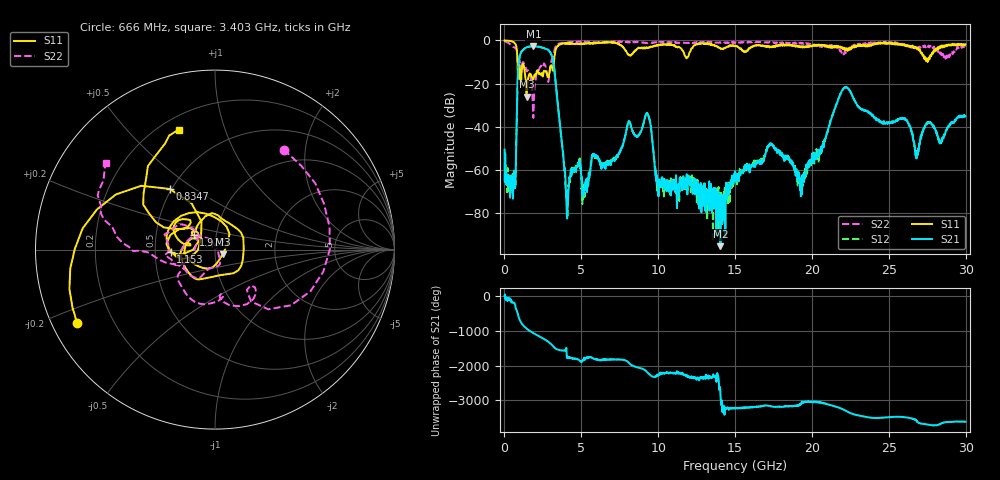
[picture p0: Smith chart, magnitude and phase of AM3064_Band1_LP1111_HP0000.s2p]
# Hz S DB R 50.0
!freq dBS11 angS11 dBS21 angS21 dBS12 angS12 dBS22 angS22
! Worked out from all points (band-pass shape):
!   1600 points, 10 MHz to 29.98 GHz, reference 50 ohm
!   highest |S21| = -2.65 dB at 1.884 GHz (marker M1); lowest = -95.4 dB at 14.05 GHz (marker M2)
!   |S21| within 3 dB of the highest: 1.07 GHz to 2.984 GHz (1.914 GHz wide, 94.4 % of centre)
!   lowest |S11| = -26.1 dB at 1.435 GHz (marker M3), VSWR 1.10, Z = 54.4 - j2.68 ohm
!   |S11| at or under -10 dB: 849 MHz to 3.217 GHz (2.368 GHz wide, 116 % of centre)
!   |S22| runs from -36.0 to -0.2 dB; largest |S21 - S12| = 0.014
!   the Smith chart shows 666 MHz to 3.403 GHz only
!   S11 on the Smith chart (normalised r, x): 666 MHz: 0.07, -0.25; 834.7 MHz: 0.49, +0.40; 1.153 GHz: 0.60, -0.01; 1.922 GHz: 0.78, +0.13; 3.403 GHz: 0.27, +0.71
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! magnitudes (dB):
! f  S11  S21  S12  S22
! 10 MHz  0.0  -50.7  -65.0  -0.2
! 666 MHz  -1.2  -64.3  -66.5  -3.4
! 834.7 MHz  -7.5  -24.9  -24.8  -7.0
! 1.153 GHz  -12.2  -4.9  -4.8  -10.8
! 1.435 GHz  -26.1  -3.2  -3.2  -14.2
! 1.884 GHz  -17.9  -2.7  -2.7  -36.0
! 1.922 GHz  -16.9  -2.7  -2.6  -25.6
! 3.009 GHz  -11.7  -5.9  -5.9  -10.9
! 3.403 GHz  -3.1  -24.9  -25.0  -2.2
! 4.04 GHz  -1.5  -76.8  -74.4  -0.9
! 5.015 GHz  -1.5  -64.4  -69.2  -0.4
! 9.269 GHz  -3.2  -33.9  -33.6  -1.3
! 10 GHz  -2.2  -66.9  -64.2  -0.9
! 14.05 GHz  -3.7  -95.4  -79.2  -1.0
! 15 GHz  -2.5  -60.8  -62.3  -1.2
! 17.27 GHz  -3.0  -48.4  -47.8  -1.0
! 19.28 GHz  -3.2  -72.3  -63.7  -1.2
! 19.99 GHz  -2.8  -55.5  -56.3  -1.8
! 22.15 GHz  -4.5  -21.9  -21.8  -5.2
! 25 GHz  -1.1  -38.0  -38.1  -1.0
! 26.81 GHz  -3.5  -52.6  -54.4  -3.7
! 29.98 GHz  -1.8  -35.3  -35.1  -2.9
